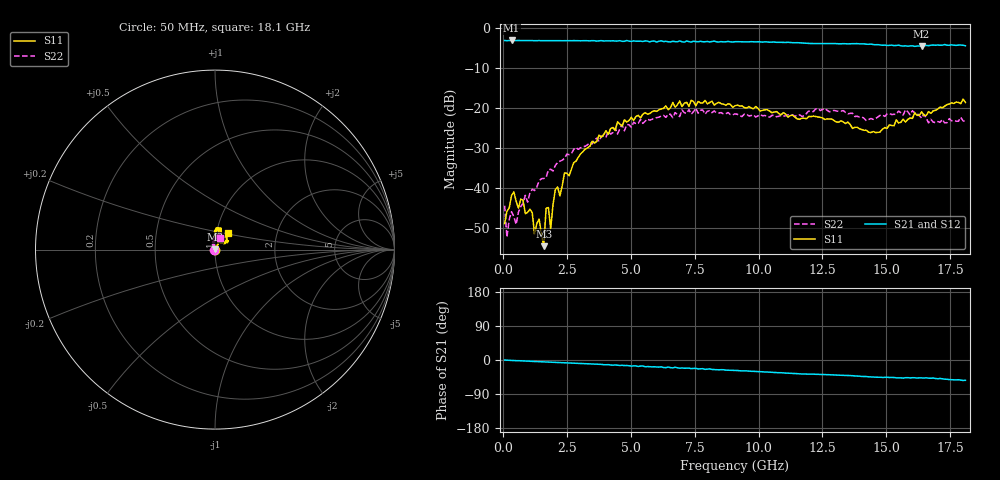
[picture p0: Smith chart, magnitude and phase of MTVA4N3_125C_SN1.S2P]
! Network Analyzer HP8720D.06.14 Serial No. US36140669
! 11 May 2005  10:13:56
! Frequency  S11  S21  S12  S22
# HZ  S  DB R 50
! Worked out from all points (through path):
!   201 points, 50 MHz to 18.1 GHz, reference 50 ohm
!   highest |S21| = -3.21 dB at 320.8 MHz (marker M1); lowest = -4.7 dB at 16.39 GHz (marker M2)
!   group delay of S21, straight-line fit = 8.25 ps
!   lowest |S11| = -54.6 dB at 1.584 GHz (marker M3), VSWR 1.00, Z = 50.1 + j0.176 ohm
!   |S11| at or under -10 dB: start of sweep to end of sweep
!   |S22| runs from -52.3 to -20.1 dB; largest |S21 - S12| = 0.027
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5e7  -48.92 -93.2  -3.21 -0.1  -3.22 -0.6  -44.45 -128.7
1.4025e8  -45.91 -131.5  -3.26 -0.5  -3.25 -1.0  -52.33 -138.8
3.2075e8  -41.94 -167.6  -3.21 -1.0  -3.23 -1.4  -45.96 -153.5
5.0125e8  -43.31 -146.2  -3.24 -1.8  -3.23 -2.1  -49.15 163.4
1.133e9  -46.25 -175.7  -3.24 -3.7  -3.25 -4.0  -40.37 133.9
1.22325e9  -51.55 172.5  -3.26 -3.9  -3.25 -4.3  -40.67 125.8
1.40375e9  -47.78 154.1  -3.24 -4.4  -3.25 -4.8  -38.17 130.0
1.58425e9  -54.56 70.3  -3.26 -5.0  -3.26 -5.3  -37.65 120.1
1.6745e9  -45.13 79.3  -3.25 -5.2  -3.26 -5.6  -37.47 122.3
1.76475e9  -44.90 107.2  -3.26 -5.5  -3.24 -5.9  -35.50 117.1
1.855e9  -50.20 93.9  -3.26 -5.8  -3.26 -6.1  -35.35 113.6
2.0355e9  -40.47 63.0  -3.26 -6.3  -3.26 -6.7  -34.43 116.5
2.216e9  -42.01 70.2  -3.27 -6.9  -3.24 -7.2  -33.35 104.5
2.3965e9  -36.27 57.6  -3.26 -7.3  -3.26 -7.8  -32.61 108.3
3.1185e9  -30.96 61.9  -3.27 -9.4  -3.29 -10.0  -29.73 115.4
4.47225e9  -23.51 63.2  -3.36 -13.7  -3.29 -13.5  -26.55 99.6
6.09675e9  -20.52 74.5  -3.39 -18.7  -3.32 -19.0  -22.35 79.7
9.075e9  -19.52 86.6  -3.52 -27.6  -3.48 -28.0  -21.53 64.6
1.21435e10  -22.09 87.8  -3.98 -37.2  -3.93 -37.7  -20.97 74.9
1.512175e10  -24.30 40.6  -4.43 -46.1  -4.31 -46.2  -21.49 77.5
1.638525e10  -21.00 33.3  -4.69 -47.2  -4.51 -47.2  -22.59 55.0
1.81e10  -18.69 51.4  -4.54 -53.6  -4.55 -54.8  -23.41 68.0
